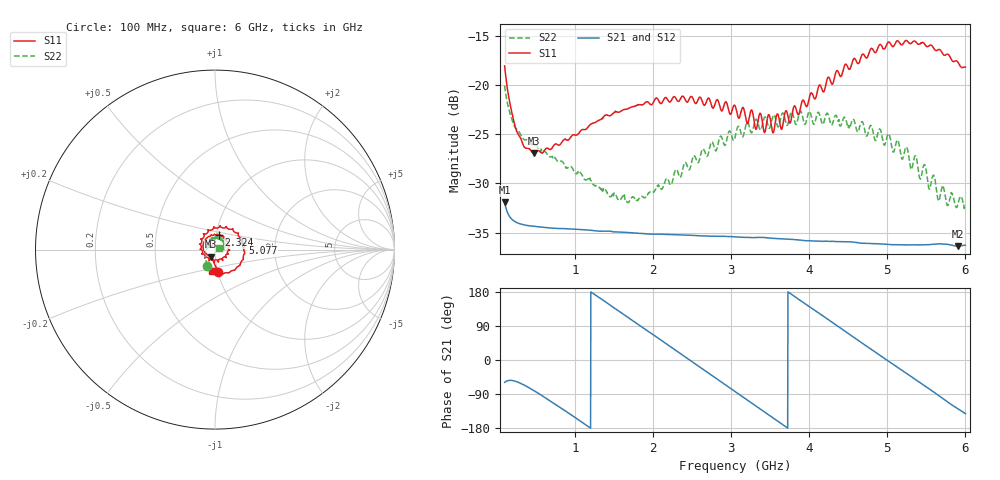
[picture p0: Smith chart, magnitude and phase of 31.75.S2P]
!Agilent Technologies,E5071C,MY46316741,A.11.02
!Date: Thu Dec 16 09:41:30 2021
!Data & Calibration Information:
!Freq	S11:SOLT4(ON)	S21:SOLT4(ON)	S12:SOLT4(ON)	S22:SOLT4(ON)
!PortZ  Port1:50+j0  Port2:50+j0
!Above PortZ is port z conversion or system Z0 setting when saving the data.
!When reading, reference impedance value at option line is always used.
# Hz S dB R 50
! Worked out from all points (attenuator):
!   1593 points, 100 MHz to 6 GHz, reference 50 ohm
!   highest |S21| = -31.92 dB at 100 MHz (marker M1); lowest = -36.4 dB at 5.907 GHz (marker M2)
!   lowest |S11| = -26.9 dB at 478 MHz (marker M3), VSWR 1.09, Z = 47.8 - j3.81 ohm
!   |S11| at or under -10 dB: start of sweep to end of sweep
!   |S22| runs from -32.6 to -20.1 dB; largest |S21 - S12| = 0.00012
!   S11 on the Smith chart (normalised r, x): 100 MHz: 1.01, -0.25; 2.324 GHz: 1.03, +0.16; 5.077 GHz: 1.35, +0.10; 6 GHz: 0.94, -0.23
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1e8  -18.08 -81.5  -31.92 -59.1  -31.92 -59.1  -20.08 -115.6
2.519472e8  -24.66 -100.6  -33.97 -57.1  -33.97 -57.1  -24.49 -155.2
4.780151e8  -26.94 -117.9  -34.36 -81.0  -34.37 -80.9  -26.16 177.0
1.085804e9  -24.57 -166.9  -34.70 -163.5  -34.70 -163.5  -29.08 145.4
1.678769e9  -22.42 138.8  -34.99 112.5  -35.00 112.5  -31.96 146.7
2.067902e9  -21.53 104.4  -35.16 57.5  -35.16 57.6  -30.15 152.4
2.323618e9  -21.68 74.7  -35.22 21.0  -35.23 21.0  -29.00 151.9
3.05e9  -22.10 -17.9  -35.44 -82.9  -35.45 -82.7  -25.36 117.2
3.539196e9  -24.87 -107.8  -35.58 -153.1  -35.59 -152.9  -23.08 92.7
4.035804e9  -20.86 160.3  -35.84 136.1  -35.84 136.3  -23.48 69.3
4.576884e9  -17.31 78.0  -35.99 58.7  -35.98 58.9  -23.62 37.0
5.017902e9  -15.64 21.7  -36.21 -3.5  -36.21 -3.4  -24.98 13.2
5.077198e9  -16.11 13.9  -36.24 -11.8  -36.22 -11.5  -26.83 10.2
5.247676e9  -15.50 -6.3  -36.25 -35.7  -36.26 -35.5  -26.32 5.4
5.303266e9  -15.79 -13.9  -36.25 -43.4  -36.25 -43.1  -28.56 4.1
5.47745e9  -15.85 -34.2  -36.24 -68.0  -36.26 -67.7  -28.10 -0.0
5.547864e9  -15.97 -44.9  -36.22 -77.8  -36.21 -77.5  -30.49 -3.6
5.592337e9  -16.26 -48.7  -36.18 -84.1  -36.20 -83.8  -29.17 0.6
5.655339e9  -16.41 -58.3  -36.14 -93.4  -36.13 -93.1  -31.79 2.5
5.71093e9  -16.85 -63.5  -36.17 -101.7  -36.17 -101.2  -30.33 2.3
5.907349e9  -17.73 -86.3  -36.38 -129.1  -36.38 -128.8  -32.05 11.9
6e9  -18.20 -97.8  -36.28 -141.7  -36.27 -141.4  -32.35 21.1
